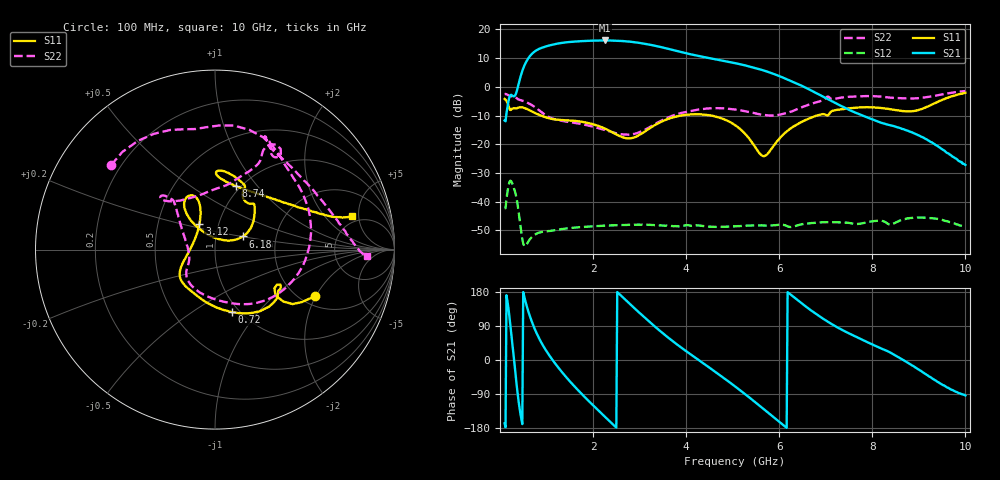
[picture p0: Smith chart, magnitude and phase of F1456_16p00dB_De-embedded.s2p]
! Integrated Device Technology
! Corporate Headquarters
! 6024 Silver Creek Valley Road
! San Jose, CA 95138  USA
! Phone:  1-408-284-8200
! Toll Free:  1-800-223-1366
! Webpage:  http://www.idt.com/
! Timing and RF Division
! 515 Groton Road, Suite 102
! Westford, MA 01886-6024
! Device:  F1456
! Description: 6-bit 0.5 dB Transmit Variable Gain Amplifier
! Frequency:  2100.0 -  2950.00 MHz
! Package:  6x6 mm Thin QFN Plastic Package: 28 pin
! State:  32
! Atten State:  16.0 dB
! Voltage:  +5.00 Volts
! Current:  217.010 mA
! Data:  The device was measured on a the F1455 evaluation board which has
!  individual transmission lines to the RF pins.  Data was collected
!  using a calibrated network analyzer.  The evaluation board was
!  de-embedded using a TRL calibration technique.
!  The reference plane is the edge of the package pin.
!  Pin  1 = CSb
!  Pin  2 = DATA
!  Pin  3 = CLK
!  Pin  4 = RSET
!  Pin  5 = GND
!  Pin  6 = RFIN  = Port 1
!  Pin  7 = GND
!  Pin  8 = NC
!  Pin  9 = NC
!  Pin 10 = NC
!  Pin 11 = NC
!  Pin 12 = NC
!  Pin 13 = NC
!  Pin 14 = /STBY
!  Pin 15 = GND
!  Pin 16 = RFOUT  = Port 2
!  Pin 17 = GND
!  Pin 18 = NC
!  Pin 19 = NC
!  Pin 20 = NC
!  Pin 21 = GND
!  Pin 22 = NC
!  Pin 23 = GND
!  Pin 24 = NC
!  Pin 25 = NC
!  Pin 26 = NC
!  Pin 27 = GND
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# GHz S dB R 50
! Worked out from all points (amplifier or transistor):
!   496 points, 100 MHz to 10 GHz, reference 50 ohm
!   highest |S21| = 16.2 dB at 2.26 GHz (marker M1)
!   |S21| within 3 dB of that: 833.2 MHz to 3.636 GHz (2.803 GHz wide, 125 % of centre)
!   unconditionally stable (mu >= 1): start of sweep to end of sweep
!   at 1.74 GHz: K = 19.91, MAG = 16.4 dB, |S12| = -48.9 dB
!   at 5.06 GHz: K = 41.81, MAG = 9.2 dB, |S12| = -48.6 dB
!   at 10 GHz: K = 352.82, MAG = -17.7 dB, |S12| = -48.9 dB
!   S11 on the Smith chart (normalised r, x): 100 MHz: 2.35, -1.98; 720 MHz: 0.92, -0.74; 3.12 GHz: 0.81, +0.24; 6.18 GHz: 1.35, +0.20; 8.74 GHz: 0.95, +0.78; 10 GHz: 4.22, +4.07
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0.1  -4.21 -25.1  -11.73 -167.2  -42.29 48.3  -2.55 140.8
0.32  -7.48 -31.7  -3.12 -19.3  -36.34 -148.1  -3.34 66.8
0.44  -7.13 -41.4  3.43 -142.2  -48.43 136.3  -4.63 38.0
0.56  -7.62 -56.8  8.61 149.1  -55.21 161.1  -5.27 10.5
0.72  -8.85 -74.9  11.98 90.0  -51.86 140.6  -6.75 -24.0
0.96  -10.50 -98.7  13.94 31.0  -50.48 95.4  -9.64 -66.9
1.18  -11.38 -115.8  14.88 -8.3  -50.02 70.3  -11.32 -93.6
1.48  -11.72 -132.2  15.60 -53.2  -49.27 45.6  -12.28 -119.3
1.76  -12.18 -143.0  15.93 -90.1  -48.86 27.4  -13.01 -134.1
2.26  -14.60 -159.6  16.16 -150.3  -48.39 0.7  -15.12 -149.7
2.64  -17.63 172.3  15.95 165.3  -48.18 -17.8  -16.60 -165.4
3.12  -15.52 121.1  14.98 110.8  -48.08 -41.6  -14.94 159.5
3.4  -12.73 110.5  14.06 80.8  -48.25 -54.7  -12.40 143.2
3.74  -10.56 109.2  12.74 47.1  -48.60 -69.0  -9.88 132.9
4.1  -9.59 114.2  11.32 14.7  -48.43 -84.6  -8.44 131.1
5.06  -13.45 129.5  8.22 -70.5  -48.59 -128.3  -7.92 136.4
5.66  -24.19 75.5  5.73 -128.9  -48.37 -162.6  -9.79 119.4
6.18  -15.29 25.3  2.51 179.0  -48.64 164.4  -8.99 82.8
6.7  -10.66 41.3  -1.38 129.5  -47.48 139.9  -5.87 64.4
8.36  -7.74 87.9  -13.29 21.4  -47.96 68.6  -3.74 62.5
8.74  -8.56 71.7  -15.15 -5.2  -45.95 61.8  -4.06 49.2
10  -2.11 13.7  -27.24 -93.6  -48.91 -23.6  -1.46 -2.6
